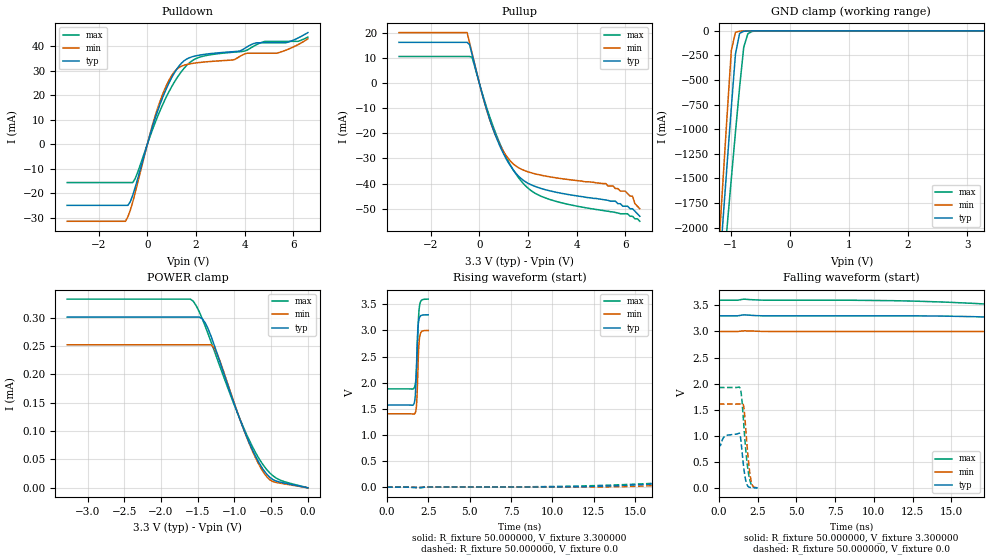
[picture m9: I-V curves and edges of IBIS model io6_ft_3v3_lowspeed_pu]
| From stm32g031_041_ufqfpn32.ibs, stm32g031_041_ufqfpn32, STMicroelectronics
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|   Model io6_ft_3v3_lowspeed_pu
[Model]  io6_ft_3v3_lowspeed_pu
Model_type I/O
Polarity   Non-Inverting
Enable   Active-Low
Vinl =   0.990000V
Vinh =   2.310000V
Vmeas =  1.650000V
Cref =   40.000000pF
Rref =   100.000000M
Vref =   0.0V
C_comp   1.290400pF   1.272500pF   1.305600pF
[Temperature Range]   25.000000   -40.000000   0.125000k
[Pullup Reference]   3.300000V   3.000000V   3.600000V
[Pulldown Reference]   0.0V   0.0V   0.0V
[POWER Clamp Reference]   3.300000V   3.000000V   3.600000V
[GND Clamp Reference]   0.0V   0.0V   0.0V
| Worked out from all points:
|   slope of the pulldown table from 0 to 0.495 V, typ, clamps not added: 31.8 ohm
|   slope of the pullup table from 0 to 0.495 V, typ, clamps not added: 30.4 ohm
|   GND clamp passes 1 mA (typ) near -0.65 V on its own axis
|   rising waveform, R_fixture 50.000000, V_fixture 3.300000: 20-80 % time 114ps typ, 109ps min, 129ps max; typ from 1.57 V to 3.3 V
|   rising waveform, R_fixture 50.000000, V_fixture 0.0: 20-80 % time 45.7ns typ, 40.3ns min, 56.9ns max; typ from 0.002 V to 1.8 V
|   falling waveform, R_fixture 50.000000, V_fixture 3.300000: 20-80 % time 40.8ns typ, 40.4ns min, 43.6ns max; typ from 3.3 V to 1.57 V
|   falling waveform, R_fixture 50.000000, V_fixture 0.0: 20-80 % time 1.61ns typ, 288ps min, 331ps max; typ from 1.8 V to 0.002 V
[Pulldown]
|Voltage   I(typ)   I(min)   I(max)
-3.3V     -25.03mA   -31.54mA   -15.7mA
-900mV    -25.03mA   -31.54mA   -15.7mA
-700mV    -23.48mA   -26.95mA   -15.7mA
-500mV    -17.69mA   -19.75mA   -14.07mA
100mV     3.479mA    3.853mA    2.862mA
500mV     15.71mA    16.96mA    13.17mA
900mV     25.22mA    26.33mA    21.66mA
1.3V      31.91mA    31.32mA    28.29mA
2.2V      36.48mA    33.43mA    35.69mA
4.1V      39.76mA    37.15mA    38.42mA
5.3V      41.43mA    37.15mA    42.02mA
6.6V      45.6mA     43.04mA    43.74mA
[Pullup]
|Voltage   I(typ)   I(min)   I(max)
-3.3V     16.16mA    20.05mA    10.53mA
-500mV    16.16mA    20.05mA    10.53mA
-400mV    15.28mA    16.06mA    10.53mA
-300mV    11.46mA    11.98mA    10.27mA
400mV     -13.51mA   -13.75mA   -12.62mA
800mV     -24.01mA   -23.65mA   -23mA
1.3V      -33.26mA   -31.25mA   -32.99mA
1.9V      -39.28mA   -34.97mA   -40.88mA
2.6V      -42.11mA   -36.79mA   -45.26mA
5.2V      -46.5mA    -40mA      -50.9mA
6.3V      -50mA      -45mA      -53mA
6.6V      -53mA      -50mA      -55mA
[GND_clamp]
|Voltage   I(typ)   I(min)   I(max)
-3.3V     -9.61A     -9.635A    -9.699A
-1.2V     -2.493A    -2.184A    -2.958A
-1.13V    -1.917A    -1.512A    -2.469A
-1.06V    -1.345A    -845.6mA   -1.983A
-990mV    -779.8mA   -200.2mA   -1.503A
-920mV    -235.5mA   -14.18mA   -1.03A
-850mV    -26.06mA   -3.338mA   -574.2mA
-780mV    -4.499mA   -1.808mA   -166.4mA
-710mV    -1.722mA   -869.6uA   -29.45mA
-640mV    -806.7uA   -283.7uA   -6.281mA
3.28V     0A         0A         0A
[POWER_clamp]
|Voltage   I(typ)   I(min)   I(max)
-3.28V    300.8uA    252uA      332.4uA
-1.6V     300.8uA    252uA      332.4uA
-1.56V    300.8uA    252uA      328.4uA
-1.44V    297.9uA    252uA      298.3uA
-1.36V    280.4uA    252uA      271.4uA
-1.28V    252.9uA    246.9uA    243.1uA
-1.2V     222.5uA    224.3uA    214.5uA
-920mV    118.6uA    118.8uA    119.5uA
-680mV    47.6uA     44.33uA    54.63uA
-560mV    24.08uA    19.48uA    32.08uA
-480mV    14.89uA    11.29uA    21.67uA
0V        0A         0A         0A
[Ramp]
| variable   typ   min   max
dV/dt_r  1.07498/45.58410n   0.96348/40.27532n   1.14311/56.84670n
dV/dt_f  1.02906/40.72304n   0.95214/40.30338n   1.02300/43.52075n
R_load = 50.000000
[Rising Waveform]
R_fixture= 50.000000
V_fixture= 3.300000
V_fixture_min= 3.000000
V_fixture_max= 3.600000
|time   V(typ)   V(min)   V(max)
0s        1.573V     1.405V     1.883V
1.542ns   1.569V     1.403V     1.88V
1.657ns   1.623V     1.402V     1.909V
1.727ns   1.834V     1.439V     2.003V
1.792ns   2.389V     1.602V     2.299V
1.852ns   2.94V      2.067V     2.806V
1.917ns   3.184V     2.655V     3.297V
1.967ns   3.248V     2.857V     3.47V
2.052ns   3.284V     2.964V     3.565V
2.492ns   3.3V       3V         3.6V
[Rising Waveform]
R_fixture= 50.000000
V_fixture= 0.0
V_fixture_min= 0.0
V_fixture_max= 0.0
|time   V(typ)   V(min)   V(max)
0s        1.56mV     1.094mV    2.417mV
11.61ns   10.68mV    3.645mV    23.48mV
17.62ns   88.61mV    52.9mV     98.96mV
44.84ns   851.3mV    812.6mV    747.3mV
54.45ns   1.091V     1.044V     978.6mV
68.47ns   1.36V      1.284V     1.26V
84.08ns   1.555V     1.442V     1.498V
105.3ns   1.69V      1.542V     1.707V
127.3ns   1.751V     1.582V     1.819V
199.4ns   1.797V     1.608V     1.925V
[Falling Waveform]
R_fixture= 50.000000
V_fixture= 3.300000
V_fixture_min= 3.000000
V_fixture_max= 3.600000
|time   V(typ)   V(min)   V(max)
0s        3.3V       3V         3.6V
14.41ns   3.295V     3V         3.565V
25.63ns   3.13V      2.935V     3.347V
33.63ns   2.914V     2.765V     3.133V
61.66ns   2.14V      2.026V     2.421V
73.67ns   1.907V     1.78V      2.211V
84.08ns   1.787V     1.641V     2.1V
102.9ns   1.683V     1.52V      1.998V
126.5ns   1.624V     1.456V     1.939V
199.4ns   1.573V     1.405V     1.883V
[Falling Waveform]
R_fixture= 50.000000
V_fixture= 0.0
V_fixture_min= 0.0
V_fixture_max= 0.0
|time   V(typ)   V(min)   V(max)
0s        1.797V     1.608V     1.925V
5.005ps   1.178V     1.608V     1.925V
10.01ps   1.056V     1.608V     1.925V
60.06ps   812.1mV    1.608V     1.925V
395.4ps   994.2mV    1.608V     1.925V
1.371ns   1.009V     1.608V     1.91V
1.602ns   394.3mV    1.554V     1.23V
1.917ns   20.42mV    489.1mV    266.2mV
2.142ns   3.955mV    63.15mV    39.1mV
2.492ns   1.56mV     1.094mV    2.417mV
